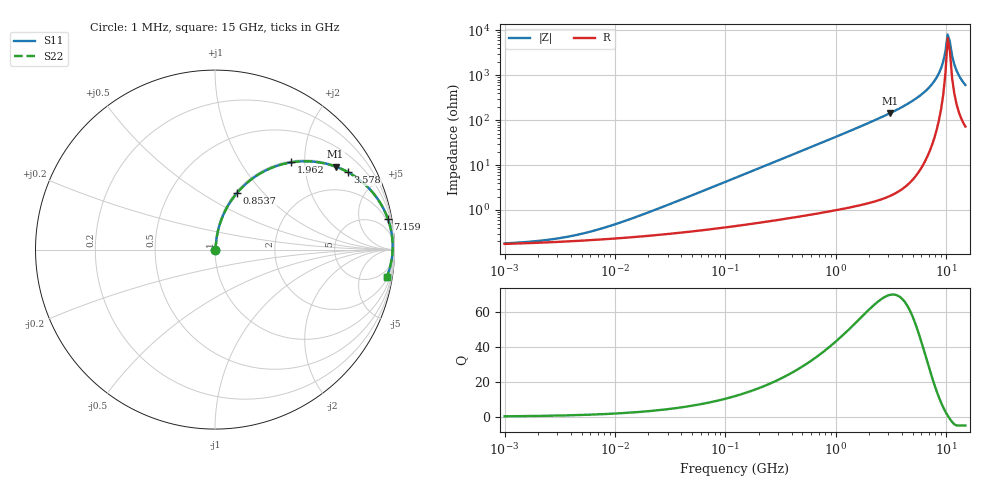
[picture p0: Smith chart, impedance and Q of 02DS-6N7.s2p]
# MHz S MA R 50
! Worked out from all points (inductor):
!   209 points, 1 MHz to 15 GHz, reference 50 ohm
!   read as one part in series: L = 6.7 nH near 19.27 MHz
!   highest Q = 69.8 at 3.115 GHz (marker M1), where L = 7.34 nH
!   self-resonance near 10.36 GHz
!   S11 on the Smith chart (normalised r, x): 1 MHz: 1.00, +0.00; 853.7 MHz: 1.02, +0.72; 1.962 GHz: 1.03, +1.71; 3.578 GHz: 1.05, +3.41; 7.159 GHz: 1, +11; 15 GHz: 2, -12
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1  0.001806 13.4  0.9982 -0.0  0.9982 -0.0  0.001806 13.4
2.40697  0.002152 28.0  0.9981 -0.1  0.9981 -0.1  0.002152 28.0
5.04322  0.002969 45.4  0.9979 -0.1  0.9979 -0.1  0.002969 45.4
25.434  0.01104 74.7  0.9971 -0.6  0.9971 -0.6  0.01104 74.7
128.269  0.05387 82.2  0.9941 -3.1  0.9941 -3.1  0.05387 82.2
617.665  0.2507 73.7  0.9604 -14.5  0.9604 -14.5  0.2507 73.7
853.679  0.3375 68.8  0.9328 -19.7  0.9328 -19.7  0.3375 68.8
1961.95  0.645 48.9  0.7536 -40.2  0.7536 -40.2  0.645 48.9
3115.02  0.8155 34.6  0.5672 -54.6  0.5672 -54.6  0.8155 34.6
3578.43  0.8571 30.2  0.503 -59.0  0.503 -59.0  0.8571 30.2
5424.87  0.9467 17.7  0.3042 -71.2  0.3042 -71.2  0.9467 17.7
7159.02  0.9781 10.0  0.1742 -77.8  0.1742 -77.8  0.9781 10.0
8224.05  0.9864 6.4  0.1109 -79.8  0.1109 -79.8  0.9864 6.4
9020.7  0.9892 3.9  0.06933 -79.1  0.06933 -79.1  0.9892 3.9
9447.52  0.9899 2.8  0.04886 -76.7  0.04886 -76.7  0.9899 2.8
9894.53  0.9901 1.6  0.02894 -69.2  0.02894 -69.2  0.9901 1.6
10362.7  0.9898 0.4  0.01219 -32.7  0.01219 -32.7  0.9898 0.4
10853  0.9889 -0.8  0.01775 51.1  0.01775 51.1  0.9889 -0.8
11366.5  0.9876 -2.0  0.03651 69.2  0.03651 69.2  0.9876 -2.0
11904.3  0.9858 -3.2  0.05657 73.8  0.05657 73.8  0.9858 -3.2
13057.5  0.9805 -5.5  0.09739 75.7  0.09739 75.7  0.9805 -5.5
15000  0.9685 -9.1  0.1591 74.1  0.1591 74.1  0.9685 -9.1
